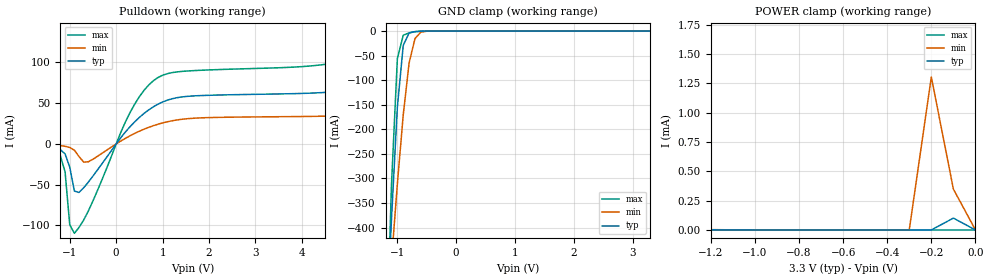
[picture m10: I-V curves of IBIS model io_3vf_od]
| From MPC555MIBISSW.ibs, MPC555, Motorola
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| io_3vf_od
[Model]   io_3vf_od
Model_type   I/O
Polarity   Non-Inverting
C_comp   6.7080e-13   6.0050e-13   7.6470e-13
| CAP models
| typical : model= typ
| maximum : model= wcs
| minimum : model= bcs
[Voltage range]   3.3v   3.0v   3.6v
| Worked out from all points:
|   slope of the pulldown table from 0 to 0.495 V, typ, clamps not added: 15.3 ohm
|   GND clamp passes 1 mA (typ) near -0.70 V on its own axis
|   POWER clamp passes 1 mA (typ) near -2.50 V on its own axis
|  typical: model = typ,  temp = 25,  vdd = 3.3
|  maximum: model = bcs,  temp = -40, vdd = 3.6
|  minimum: model = wcs,  temp = 150, vdd = 3.0
[Pulldown]
|  Voltage   I(typ)   I(min)   I(max)
-3.3V     -830uA     -300uA     -1.4mA
-1.3V     -4.911mA   -1.631mA   -8.96mA
-1.1V     -12.31mA   -2.871mA   -34.49mA
-1V       -28.48mA   -4.35mA    -99.26mA
-900mV    -57.85mA   -7.714mA   -109.7mA
-600mV    -46.97mA   -21.95mA   -82.43mA
300mV     21.25mA    10.05mA    38.67mA
900mV     48.81mA    24.2mA     81.5mA
5.6V      71.39mA    38.01mA    114mA
5.9V      86.24mA    88.86mA    122.6mA
6.1V      164.9mA    151mA      195.5mA
6.6V      416.3mA    321.6mA    530.3mA
[GND_clamp]
-3.3V     -6.942A    -4.403A    -10.42A
-1.2V     -648.1mA   -632.8mA   -705.4mA
-1.1V     -383mA     -468.1mA   -313.1mA
-1V       -154.9mA   -311.4mA   -56.14mA
-900mV    -29.19mA   -170.4mA   -8.377mA
-800mV    -3.643mA   -64.63mA   -3.772mA
-700mV    -1.021mA   -15.21mA   -1.258mA
-600mV    -239.5uA   -2.066mA   -170.3uA
-400mV    -1.896uA   -47.44uA   -129.1nA
3.3V      52.74pA    15.4nA     1.967nA
[POWER_clamp]
-3.3V     326.4mA    252.4mA    344.4mA
-2.9V     131.9mA    17.75mA    208.9mA
-2.7V     43.4mA     113.1uA    142.8mA
-2.6V     10.66mA    99.3uA     110.6mA
-2.4V     64.47uA    81.32uA    49.87mA
-2.2V     36.14uA    64.17uA    6.272mA
-2V       27.04uA    47.68uA    93.46uA
-1.9V     22.74uA    39.53uA    18.75uA
-300mV    62.04pA    51.07nA    15.43nA
-200mV    65.85pA    1.303mA    15.55nA
-100mV    101uA      348.4uA    16.09nA
0V        45.46pA    40.86pA    12.46nA
| RAMP models
| typical dv/dt : model=typ, temp=25
| maximum dv/dt : model=bcs, temp=-40
| minimum dv/dt : model=wcs, temp=150
|		 typ   min   max
[Ramp]
dV/dt_r	 1.52577/3.23061E-10   0.941414/3.884E-10   2.25156/1.85321E-10
dV/dt_f  1.52577/3.02278E-10   0.941414/4.27607E-10   2.25156/1.73518E-10
